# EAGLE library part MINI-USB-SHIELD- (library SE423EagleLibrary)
MINI USB Connector Source: http://www.hirose.co.jp/cataloge_hp/e24000019.pdf
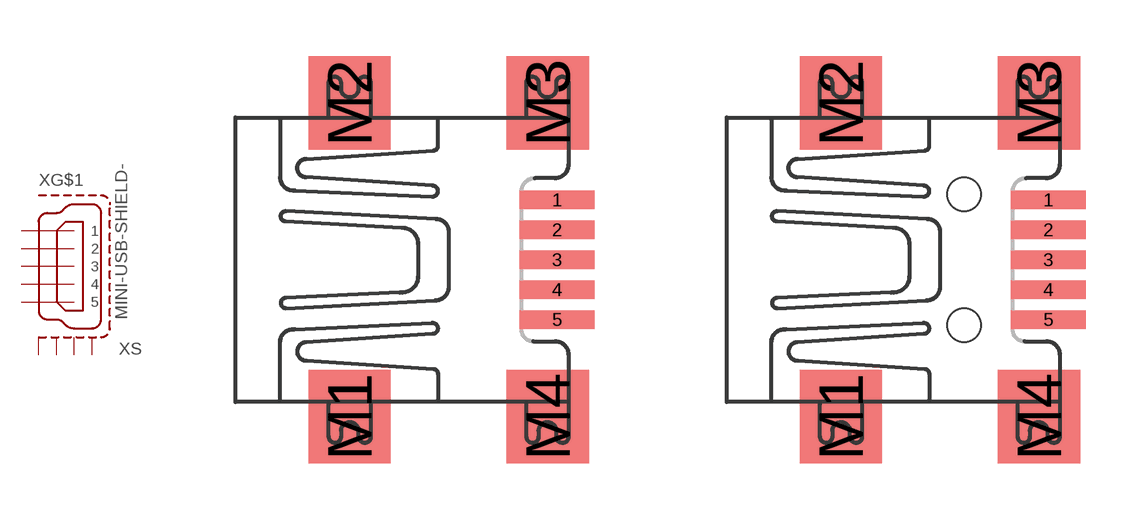
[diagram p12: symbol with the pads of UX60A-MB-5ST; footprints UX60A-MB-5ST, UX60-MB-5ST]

Designator prefix X; gates G$1=MINI-USB S=USB-SHIELD

## MINI-USB-SHIELD-UX60A-MB-5ST (OC_FARNELL: unknown; OC_NEWARK: unknown)  [UX60A-MB-5ST]
1  G$1:1  in
2  G$1:2  in
3  G$1:3  in
4  G$1:4  in
5  G$1:5  in
M1  S:S1  pas
M2  S:S2  pas
M3  S:S3  pas
M4  S:S4  pas

## MINI-USB-SHIELD-UX60-MB-5ST (OC_FARNELL: unknown; OC_NEWARK: unknown)  [UX60-MB-5ST]
Pads as for UX60A-MB-5ST

## MINI-USB-SHIELD-UX60-MB-5S8 (OC_FARNELL: unknown; OC_NEWARK: unknown)  [UX60-MB-5S8]
Pads as for UX60A-MB-5ST

## Footprint UX60A-MB-5ST (pad centres in mm)
MINI USB Connector HI-SPEED Certified Metal Shield SMT Type Without Positioning Post Source: http://www.hirose.co.jp/cataloge_hp/e24000019.pdf
smd 2 x 0.5: 1 2.25,1.6; 2 2.25,0.8; 3 2.25,0; 4 2.25,-0.8; 5 2.25,-1.6
smd 2.2 x 2.5: M1 -3.3,-4.2; M2 -3.3,4.2; M3 2,4.2; M4 2,-4.2

## Footprint UX60-MB-5ST (pad centres in mm)
MINI USB Connector HI-SPEED Certified Metal Shield SMT Type With Positioning Post Source: http://www.hirose.co.jp/cataloge_hp/e24000019.pdf
smd 2 x 0.5: 1 2.25,1.6; 2 2.25,0.8; 3 2.25,0; 4 2.25,-0.8; 5 2.25,-1.6
smd 2.2 x 2.5: M1 -3.3,-4.2; M2 -3.3,4.2; M3 2,4.2; M4 2,-4.2
hole 0.9 at 0,-1.75
hole 0.9 at 0,1.75

## Footprint UX60-MB-5S8 (pad centres in mm)
MINI USB Connector HI-SPEED Certified Metal Shield Dip Type With Positioning Post Source: http://www.hirose.co.jp/cataloge_hp/e24000019.pdf
smd 2 x 0.5: 1 8.65,1.6; 2 8.65,0.8; 3 8.65,0; 4 8.65,-0.8; 5 8.65,-1.6
drill 0.8 long: M1 3.1,-3.65; M2 3.1,3.65; M3 8.4,3.65; M4 8.4,-3.65
hole 0.9 at 6.4,-1.75
hole 0.9 at 6.4,1.75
